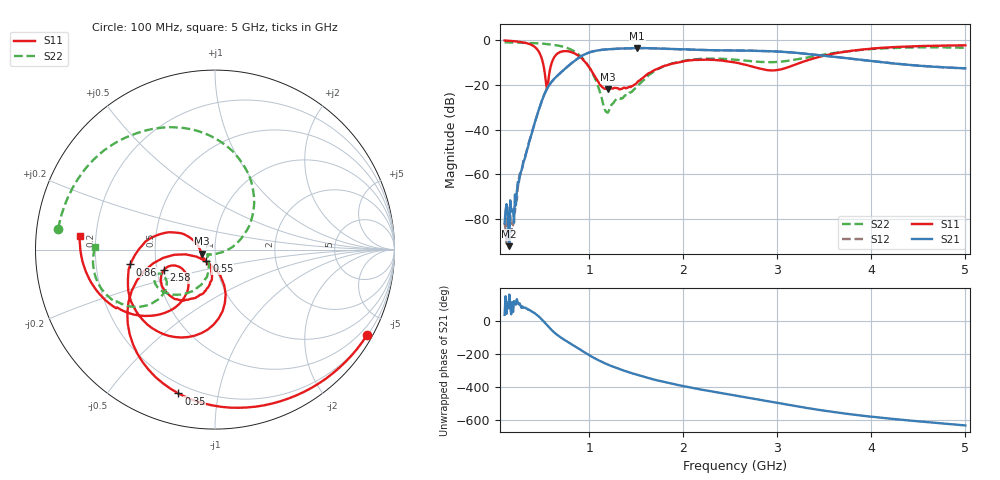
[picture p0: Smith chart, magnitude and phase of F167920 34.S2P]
!  2-Port S-parameters saved by WinCal
! VAR MeasName=S-Parameters (CALIBRATED_DATA) read from VNA (N5242A)
! VAR MeasDate=2016-11-22 9:56:54
! VAR NAME=F167920 34
! VAR FILENAME=F167920 34.S2P
! VAR DATE=2016-11-22 9:56:54
! VAR PHYS_PORTS=1,2
# Hz S DB R 50
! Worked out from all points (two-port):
!   491 points, 100 MHz to 5 GHz, reference 50 ohm
!   highest |S21| = -3.64 dB at 1.51 GHz (marker M1); lowest = -92.0 dB at 150 MHz (marker M2)
!   |S21| within 3 dB of the highest: 943 MHz to 3.412 GHz (2.469 GHz wide, 113 % of centre)
!   lowest |S11| = -22.1 dB at 1.2 GHz (marker M3), VSWR 1.17, Z = 43 - j1.94 ohm
!   |S11| at or under -10 dB: 505.9 MHz to 603.2 MHz (97.34 MHz wide, 17.6 % of centre); 959.1 MHz to 1.953 GHz (994.2 MHz wide, 68.3 % of centre); 2.541 GHz to 3.257 GHz (716.3 MHz wide, 24.7 % of centre)
!   |S22| runs from -32.4 to -1.1 dB; largest |S21 - S12| = 0.0018
!   S11 on the Smith chart (normalised r, x): 100 MHz: 0.22, -3.82; 350 MHz: 0.15, -0.77; 550 MHz: 0.90, -0.12; 860 MHz: 0.35, -0.08; 2.58 GHz: 0.55, -0.14; 5 GHz: 0.14, +0.05
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1e8  -0.25 -29.3  -81.88 36.6  -81.49 75.9  -1.10 172.4
1.5e8  -0.40 -43.6  -92.03 159.7  -78.25 20.5  -1.13 168.6
1.9e8  -0.54 -55.1  -75.65 53.9  -82.68 98.3  -1.16 165.5
2.6e8  -0.88 -75.5  -61.55 106.1  -59.71 101.6  -1.22 159.9
3.5e8  -1.65 -104.3  -47.59 67.7  -47.54 70.9  -1.33 152.2
4.5e8  -4.41 -144.3  -33.02 33.4  -32.99 33.1  -1.52 142.4
5.5e8  -21.79 -126.3  -21.89 -25.3  -21.87 -25.2  -1.87 131.1
6.1e8  -9.23 -83.0  -18.19 -60.8  -18.18 -60.7  -2.16 123.4
6.8e8  -5.61 -110.8  -15.24 -93.3  -15.23 -93.2  -2.64 112.9
8.6e8  -6.39 -170.0  -8.81 -158.5  -8.80 -158.4  -5.63 75.1
9.2e8  -8.16 173.5  -7.14 -179.4  -7.13 -179.5  -7.80 59.0
1.03e9  -14.25 153.6  -5.21 142.3  -5.21 142.3  -14.48 28.5
1.2e9  -22.10 -163.3  -4.16 94.8  -4.15 94.8  -32.36 -102.9
1.51e9  -18.92 -100.1  -3.64 33.4  -3.64 33.4  -20.94 -111.6
1.74e9  -12.58 -102.9  -3.86 -2.4  -3.85 -2.5  -12.80 -114.2
2.12e9  -8.95 -131.6  -4.39 -48.6  -4.39 -48.6  -8.66 -139.4
2.55e9  -10.06 -157.3  -4.72 -91.7  -4.72 -91.7  -8.83 -156.4
2.58e9  -10.30 -158.4  -4.73 -94.6  -4.73 -94.7  -8.94 -156.8
2.96e9  -13.62 -142.2  -5.11 -132.6  -5.11 -132.7  -9.91 -148.9
3.37e9  -8.46 -123.9  -6.45 -172.5  -6.44 -172.5  -7.45 -138.8
4.19e9  -3.33 -157.3  -10.30 128.6  -10.29 128.4  -3.67 -157.7
5e9  -2.42 174.2  -12.67 86.8  -12.66 86.5  -3.51 178.8
